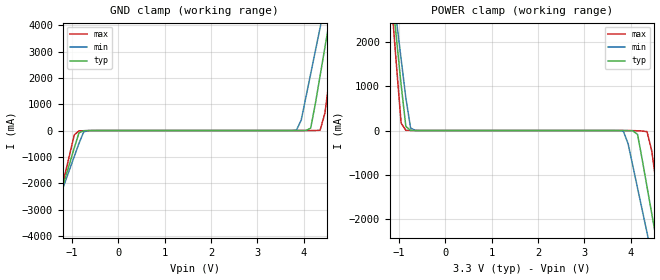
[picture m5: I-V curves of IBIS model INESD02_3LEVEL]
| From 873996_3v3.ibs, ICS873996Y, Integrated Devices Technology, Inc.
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[Model]   INESD02_3LEVEL
Model_type   Input
Polarity   Non-Inverting
Vinl = 0.8V
Vinh = 2.0V
|   typ   min   max
C_comp   2pF   1.5pF   2.5pF
|   typ   min   max
[Voltage range]  3.3V   3.15V   3.45V
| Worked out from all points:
|   GND clamp passes 1 mA (typ) near -0.58 V on its own axis
|   POWER clamp passes 1 mA (typ) near -0.67 V on its own axis
[GND_clamp]
|Voltage   I(typ)   I(min)   I(max)
-3.3V     -14.52A    -12.53A    -17.87A
-1.565V   -4.277A    -3.994A    -4.784A
-1.463V   -3.675A    -3.492A    -4.014A
-952.6mV  -663.5mA   -987.5mA   -164.6mA
-850.5mV  -87.71mA   -487.7mA   -16.13mA
-646.4mV  -2.015mA   -2.785mA   -4.233mA
3.844V    146.5uA    16.49mA    95.36uA
4.151V    91.35mA    2.153A     498.3uA
4.355V    2.088A     3.911A     12.11mA
4.559V    4.201A     5.67A      2.008A
4.763V    6.316A     7.43A      4.712A
6.6V      25.37A     23.29A     29.07A
[POWER_clamp]
|Voltage   I(typ)   I(min)   I(max)
-3.3V     25.37A     21.86A     31.26A
-1.157V   3.144A     3.369A     2.842A
-1.055V   2.088A     2.49A      1.49A
-952.6mV  1.032A     1.611A     168mA
-850.5mV  91.35mA    733.6mA    4.758mA
-646.4mV  371.7uA    2.384mA    280.7uA
3.844V    -520.5uA   -15.97mA   -109.2uA
4.151V    -87.71mA   -1.296A    -5.994mA
4.355V    -1.265A    -2.298A    -23.92mA
4.559V    -2.47A     -3.3A      -1.229A
4.763V    -3.675A    -4.303A    -2.769A
6.6V      -14.52A    -13.34A    -16.63A
